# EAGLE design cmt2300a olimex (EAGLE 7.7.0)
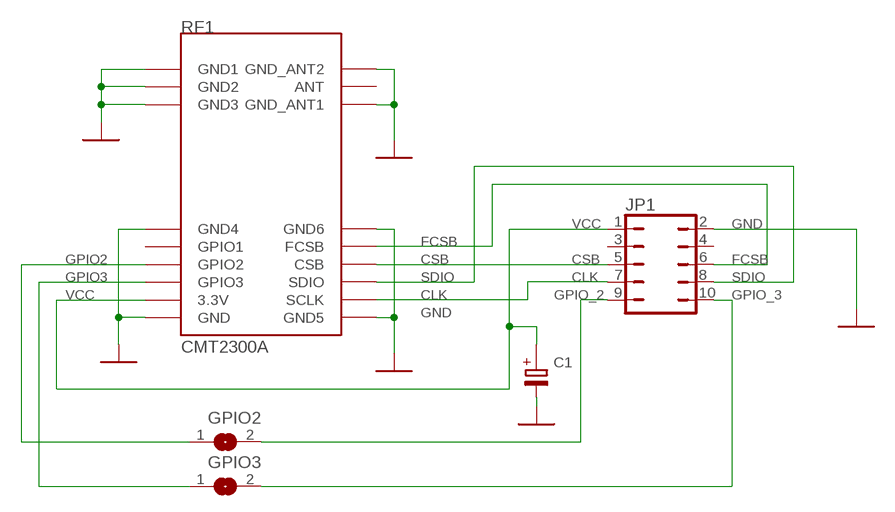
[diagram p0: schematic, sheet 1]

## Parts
C1  S470µ/16  [EB10D]
GPIO2  SJ  [SJ]
GPIO3  SJ  [SJ]
JP1  JP5Q_OT  [JP5Q_OT]
RF1  CMT2300A  [CMT2300A]

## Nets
CLK: JP1.7 RF1.SCLK
CSB: JP1.5 RF1.CSB
FCSB: JP1.6 RF1.FCSB
GND: C1.- JP1.2 RF1.GND RF1.GND1 RF1.GND2 RF1.GND3 RF1.GND4 RF1.GND5 RF1.GND6 RF1.GND_ANT1 RF1.GND_ANT2
GPIO2: GPIO2.1 RF1.GPIO2
GPIO3: GPIO3.1 RF1.GPIO3
GPIO_2: GPIO2.2 JP1.9
GPIO_3: GPIO3.2 JP1.10
SDIO: JP1.8 RF1.SDIO
VCC: C1.+ JP1.1 RF1.3.3V
Unconnected: JP1.3 JP1.4 RF1.ANT RF1.GPIO1

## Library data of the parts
C1 = 5elko:S470µ/16
GPIO2 GPIO3 = jumper_fs:SJ: SMD solder JUMPER
JP1 = jumper_fs:JP5Q: JUMPER
RF1 = cmt2300a:CMT2300A

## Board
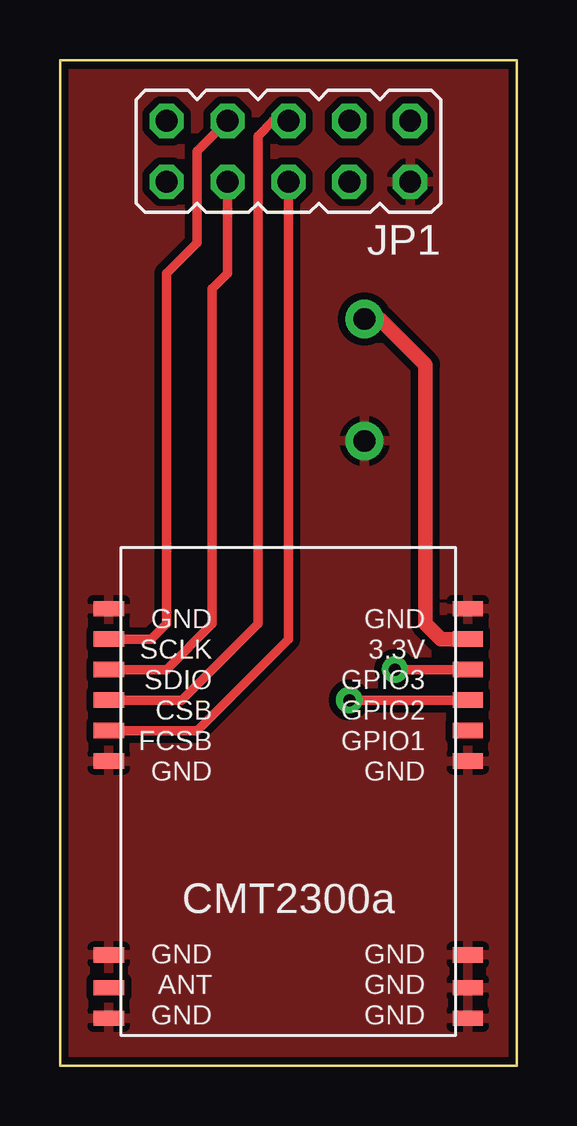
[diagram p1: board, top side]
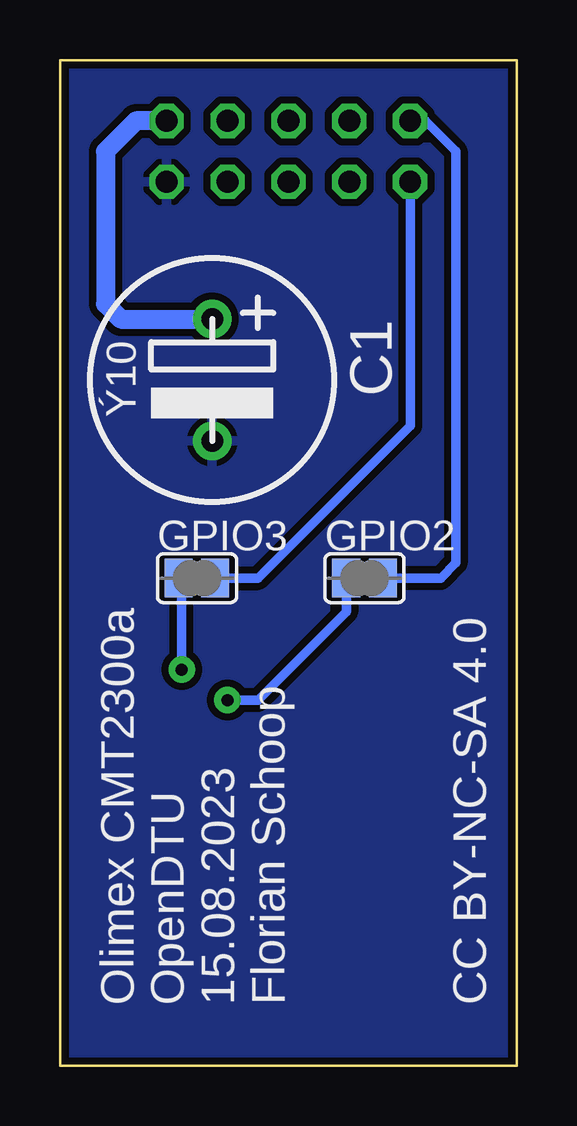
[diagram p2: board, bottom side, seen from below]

Size 19.05 x 41.91 mm. Coordinates in mm from the lower left corner, seen from the top.
Outline: 0,0 0,41.91 19.05,41.91 19.05,0 0,0
Copper layers (1*16): Component 0.035mm / dielectric 1.5mm / Solder 0.035mm
Design rules "default *": minimum track width 10mil, minimum drill 24mil, track to track 8mil, track to pad 8mil, pad to pad 8mil, via to via 8mil, smd to smd 8mil, copper to edge 8mil, drill to drill 8mil, minimum pad ring 10mil, minimum via ring 8mil, stop-mask expansion 4mil, vias tented up to drill 25mil, thermal gap 10mil

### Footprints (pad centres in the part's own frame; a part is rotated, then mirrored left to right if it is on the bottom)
EB10D = drill 0.9 pad 1.6: + -2.54,0; - 2.54,0
SJ = smd 1.168 x 1.6: 1 -0.762,0; 2 0.762,0
JP5Q_OT = drill 0.914 octagon: 1 -5.08,-1.27; 2 -5.08,1.27; 3 -2.54,-1.27; 4 -2.54,1.27; 5 0,-1.27; 6 0,1.27; 7 2.54,-1.27; 8 2.54,1.27; 9 5.08,-1.27; 10 5.08,1.27
CMT2300A = smd 1.27 x 0.635: 3.3V -0.5,2.54; ANT 14.47,17.07; CSB 14.47,5.08; FCSB 14.47,6.35; GND -0.5,1.27; GND1 -0.5,18.34; GND2 -0.5,17.07; GND3 -0.5,15.7; GND4 -0.5,7.62; GND5 14.47,1.27; GND6 14.47,7.62; GND_ANT1 14.47,15.7; GND_ANT2 14.47,18.34; GPIO1 -0.5,6.35; GPIO2 -0.5,5.08; GPIO3 -0.5,3.81; SCLK 14.47,2.54; SDIO 14.47,3.81

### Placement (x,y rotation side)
C1  12.7,28.57 270 bottom
GPIO2  6.35,20.32 0 bottom
GPIO3  13.33,20.32 0 bottom
JP1  9.53,38.1 180 top
RF1  16.51,20.32 180 top

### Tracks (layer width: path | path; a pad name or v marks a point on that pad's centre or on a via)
CLK
  Component 0.4: RF1.SCLK 3.81,17.78 4.45,18.41 4.45,33.02 5.71,34.29 5.71,38.1 JP1.7
CSB
  Component 0.4: JP1.5 8.89,39.37 8.25,38.73 8.25,18.41 5.08,15.24 RF1.CSB
FCSB
  Component 0.4: RF1.FCSB 5.71,13.97 9.53,17.78 JP1.6
GND
  pour Solder (isolate 0.3): 0,41.91 19.05,41.91 19.05,0 0,0
  pour Component (isolate 0.3): 0,41.91 19.05,41.91 19.05,0 0,0
GPIO2  (via drill 0.5 pad 1.1)
  Component 0.4: v12.06,15.24 RF1.GPIO2
  Solder 0.4: GPIO2.1 7.11,18.92 10.79,15.24 v12.06,15.24
GPIO3  (via drill 0.5 pad 1.1)
  Component 0.4: RF1.GPIO3 v13.97,16.51
  Solder 0.4: v13.97,16.51 13.97,20.19 GPIO3.1
GPIO_2
  Solder 0.4: JP1.9 3.81,39.37 2.54,38.1 2.54,20.95 3.17,20.32 GPIO2.2
GPIO_3
  Solder 0.4: GPIO3.2 10.79,20.32 4.45,26.67 JP1.10
SDIO
  Component 0.4: RF1.SDIO 4.45,16.51 6.35,18.41 6.35,32.38 6.99,33.02 JP1.8
VCC
  Component 0.6: RF1.3.3V 15.88,17.78 15.24,18.41 15.24,29.21 13.33,31.11 C1.+
  Solder 0.8: JP1.1 15.88,39.37 17.14,38.1 17.14,31.75 16.51,31.11 C1.+

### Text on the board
bNames: Olimex CMT2300a / OpenDTU / 15.08.2023 / Florian Schoop / / / / CC BY-NC-SA 4.0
